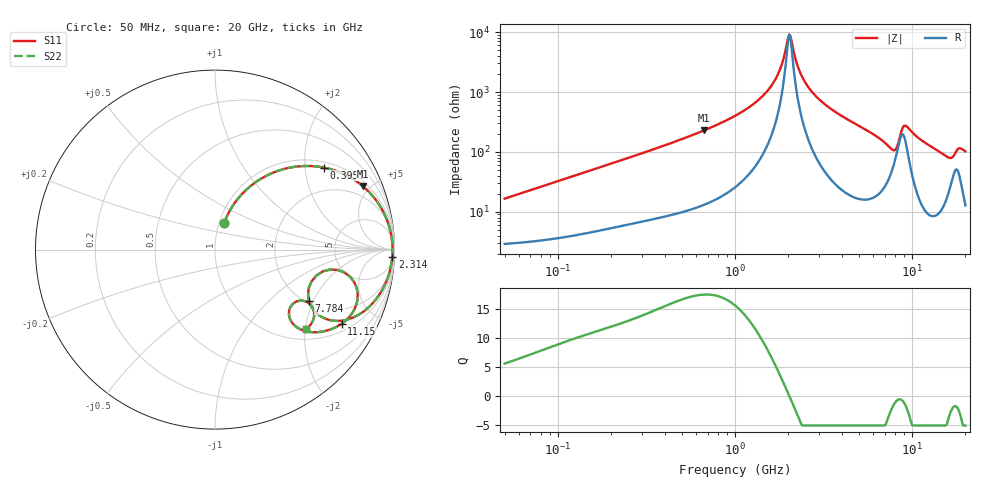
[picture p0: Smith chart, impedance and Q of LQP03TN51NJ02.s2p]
!Murata Part Number: LQP03TN51NJ02
!These Parameters are Measured in Series Mode Connection
!  o--[Z]--o
!Port1  Port2
!  o-------o
!Freq. Start=50[MHz] Stop=20[GHz], 401[Steps]
# Hz S RI R 50
!Freq.(Hz) S11(Real) S11(Imag) S21(Real) S21(Imag) S12(Real) S12(Imag) S22(Real) S22(Imag)
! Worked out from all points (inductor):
!   401 points, 50 MHz to 20 GHz, reference 50 ohm
!   read as one part in series: L = 51.6 nH near 51.52 MHz
!   highest Q = 17.5 at 667.4 MHz (marker M1), where L = 54.2 nH
!   self-resonance near 2.022 GHz
!   S11 on the Smith chart (normalised r, x): 50 MHz: 1.06, +0.33; 395.1 MHz: 1.16, +2.53; 2.314 GHz: 12, -44; 7.784 GHz: 2.08, -1.86; 11.15 GHz: 1.29, -3.20; 20 GHz: 1.26, -2.03
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5e7  0.052 0.1502  0.948 -0.1502  0.948 -0.1502  0.052 0.1502
1.364002e8  0.1839 0.342  0.8161 -0.342  0.8161 -0.342  0.1839 0.342
3.721004e8  0.5803 0.4614  0.4197 -0.4614  0.4197 -0.4614  0.5803 0.4614
3.95076e8  0.6087 0.4566  0.3913 -0.4566  0.3913 -0.4566  0.6087 0.4566
6.673612e8  0.8248 0.3526  0.1752 -0.3526  0.1752 -0.3526  0.8248 0.3526
1e9  0.9282 0.2282  0.0718 -0.2282  0.0718 -0.2282  0.9282 0.2282
1.590961e9  0.9823 0.0782  0.0177 -0.0782  0.0177 -0.0782  0.9823 0.0782
1.793498e9  0.9874 0.0397  0.0126 -0.0397  0.0126 -0.0397  0.9874 0.0397
2.021818e9  0.9893 0.0013  0.0107 -0.0013  0.0107 -0.0013  0.9893 0.0013
2.083303e9  0.9892 -0.00834  0.0108 0.00834  0.0108 0.00834  0.9892 -0.00834
2.313601e9  0.9875 -0.0423  0.0125 0.0423  0.0125 0.0423  0.9875 -0.0423
2.728004e9  0.9796 -0.0964  0.0204 0.0964  0.0204 0.0964  0.9796 -0.0964
5.194772e9  0.8528 -0.3244  0.1472 0.3244  0.1472 0.3244  0.8528 -0.3244
7.442007e9  0.5711 -0.3588  0.4289 0.3588  0.4289 0.3588  0.5711 -0.3588
7.784049e9  0.5241 -0.2877  0.4759 0.2877  0.4759 0.2877  0.5241 -0.2877
8.389408e9  0.6001 -0.1219  0.3999 0.1219  0.3999 0.1219  0.6001 -0.1219
9.041845e9  0.7705 -0.1735  0.2295 0.1735  0.2295 0.1735  0.7705 -0.1735
1.115139e10  0.7048 -0.4135  0.2952 0.4135  0.2952 0.4135  0.7048 -0.4135
1.375312e10  0.5361 -0.4596  0.4639 0.4596  0.4639 0.4596  0.5361 -0.4596
1.597544e10  0.4168 -0.384  0.5832 0.384  0.5832 0.384  0.4168 -0.384
1.747767e10  0.48 -0.2833  0.52 0.2833  0.52 0.2833  0.48 -0.2833
2e10  0.5094 -0.4409  0.4906 0.4409  0.4906 0.4409  0.5094 -0.4409
